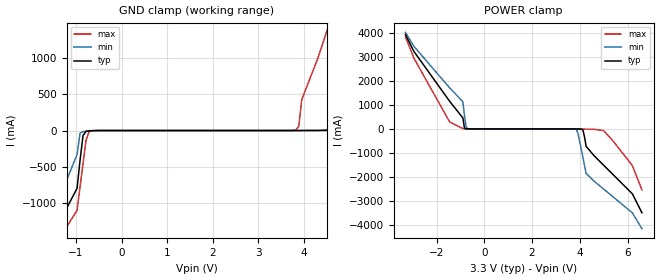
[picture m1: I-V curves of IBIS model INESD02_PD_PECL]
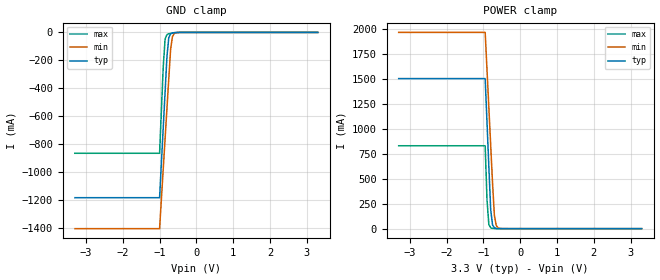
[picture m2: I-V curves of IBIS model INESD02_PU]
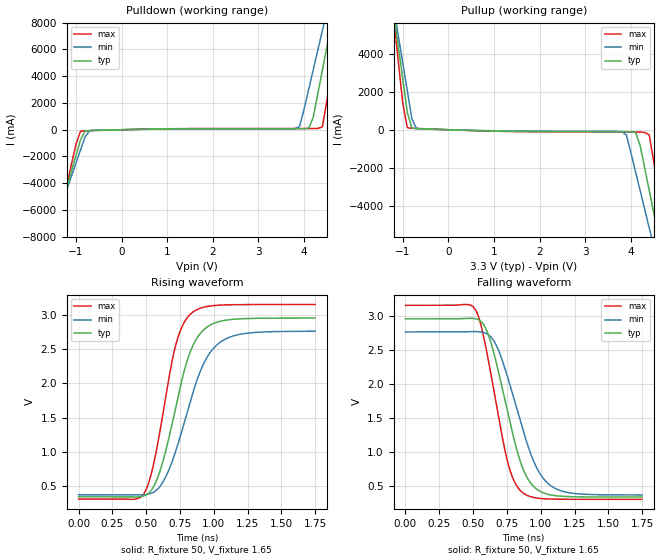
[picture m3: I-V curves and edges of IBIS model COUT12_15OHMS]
|   This file is an IBIS representation of the   |
|   Integrated Devices Technology, Inc.   |
|   ICS830584I   |
|   LOW SKEW, PCI-X 1-TO-4 FANOUT BUFFER   |
[IBIS Ver]   4.1
[File name]   830584i_3v3.ibs
[File Rev]   1.0
[Date]   2 Jun 2009 | Last modified
|   Jan  4 2007 | Generated
[Source]   Originated at Integrated Devices Technology, Inc.
[Disclaimer]
IDT hereby grants the user of this IBIS model a non-exclusive,
nontransferable license to use this IBIS model under the following terms.
Before using this IBIS model, the user should read this license.
If the user does not accept these terms,  the IBIS model should be
returned to IDT within 30 days.
   The user is granted this license only to use the IBIS model and
is not granted rights to sell, load, rent, lease or license the IBIS
model in whole or in part, or in modified form to anyone other than
user. User may modify the IBIS model to suit its specific
applications but rights to derivative works and such modifications
shall belong to IDT.
   This IBIS model is provided on an "AS IS" basis and IDT makes
absolutely no warranty with respect to the information contained
herein. IDT DISCLAIMS AND CUSTOMER WAIVES ALL WARRANTIES, EXPRESS
OR IMPLIED, INCLUDING WARRANTIES OF MERCHANTABILITY OR FITNESS FOR
A PARTICULAR PURPOSE. The entire risk as to quality and performance
is with the Customer. ACCORDINGLY, IN NO EVENT SHALL THE COMPANY BE
LIABLE FOR ANY DAMAGES, WHETHER IN CONTRACT OR TORT,INCLUDING ANY
LOST PROFITS OR OTHER INCIDENTAL, CONSEQUENTIAL, EXEMPLARY, OR
PUNITIVE DAMAGES ARISING OUT OF THE USE OR APPLICATION OF THE IBIS
model provided in this package. Further, IDT reserves the right to
make changes without notice to any product herein to improve
reliability, function, or design. IDT does not convey any license
under patent rights or any other intellectual property rights,
including those of third parties.
   IDT is not obligated to provide maintenance or support
for the licensed IBIS model.
[Copyright]   Copyright 2006 by Integrated Device Technology, Inc.
[Component]   ICS830584I
[Manufacturer] Integrated Devices Technology, Inc.
[Package]
|TSSOP 8 Lead
|   typ   min   max
R_pkg   52.5m   48.8m   56.2m
L_pkg   1.381nH   1.275nH   1.486nH
C_pkg   0.236pF   0.230pF   0.242pF
[Pin] signal_name  model_name   R_pin   L_pin   C_pin
1   CLKIN   INESD02_PD_PECL   56.2m   1.486n   0.242p
2   OE   INESD02_PU   48.8m   1.275n   0.230p
3   Q0   COUT12_15OHMS   48.8m   1.275n   0.230p
4   GND   GND   56.2m   1.468n   0.242p
5   Q1   COUT12_15OHMS   56.2m   1.486n   0.242p
6   VDD   POWER   48.8m   1.275n   0.230p
7   Q2   COUT12_15OHMS   48.8m   1.275n   0.230p
8   Q3   COUT12_15OHMS   56.2m   1.468n   0.242p
| Models and submodels in the file (3): INESD02_PD_PECL (Input), INESD02_PU (Input), COUT12_15OHMS (Output)
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[Model]   INESD02_PD_PECL
Model_type  Input
Polarity   Non-Inverting
Vinl = 0.8V
Vinh = 2.0V
|   typ   min   max
C_comp   2pF   1.5pF   2.5pF
|   typ   min   max
[Voltage range]  3.3V   3.15V   3.45V
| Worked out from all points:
|   GND clamp passes 1 mA (typ) near -0.59 V on its own axis
|   POWER clamp passes 1 mA (typ) near -0.70 V on its own axis
[GND_clamp]
-3.3V     -3.894A    -4.294A    -3.674A
-1.6V     -1.569A    -1.322A    -1.74A
-974.8mV  -794.1mA   -331.5mA   -1.096A
-843.4mV  -68.33mA   -15.34mA   -452.9mA
-646.5mV  -1.912mA   -4.151mA   -2.665mA
3.818V    89.38uA    70.49uA    7.198mA
3.95V     342.2uA    75.94uA    423.8mA
4.6V      7.437mA    165.5uA    1.553A
4.9V      78.32mA    440.9uA    2.118A
5.5V      1.293A     2.769mA    3.249A
6.25V     2.651A     112.4mA    4.38A
6.6V      3.331A     896.1mA    4.946A
[POWER_clamp]
-3.3V     3.923A     4.017A     3.838A
-2.95V    3.23A      3.44A      2.951A
-1.45V    1.149A     1.709A     289.6mA
-896.9mV  456.5mA    1.133A     15.4mA
-762.9mV  4.223mA    91.07mA    1.486mA
-695.9mV  792.2uA    10.73mA    555.6uA
3.861V    -556.7uA   -26.14mA   -39.45uA
4.129V    -41.85mA   -1.19A     -4.904mA
4.263V    -724.2mA   -1.847A    -12.04mA
5V        -1.514A    -2.505A    -71.38mA
6.2V      -2.701A    -3.492A    -1.525A
6.6V      -3.492A    -4.151A    -2.536A
[Model]   INESD02_PU
Model_type   Input
Polarity   Non-Inverting
Vinl = 0.80V
Vinh = 2.0V
|   typ   min   max
C_comp   2pF   1.5pF   2.5pF
|   typ   min   max
[Voltage range]  3.3V   3.15V   3.45V
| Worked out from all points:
|   GND clamp passes 1 mA (typ) near -0.56 V on its own axis
|   POWER clamp passes 1 mA (typ) near -0.61 V on its own axis
[GND_clamp]
|Voltage   I(typ)   I(min)   I(max)
-3.3V     -1.184A    -1.405A    -865.6mA
-1V       -1.184A    -1.405A    -865.6mA
-900mV    -678.5mA   -975.1mA   -244.1mA
-850mV    -426.2mA   -760.2mA   -46.92mA
-800mV    -174mA     -545.4mA   -16.17mA
-750mV    -37.03mA   -330.8mA   -9.981mA
-700mV    -9.767mA   -120.3mA   -7.122mA
-650mV    -3.616mA   -29.78mA   -4.922mA
-600mV    -1.7mA     -7.594mA   -3.115mA
-400mV    -123.9uA   -126uA     -173.9uA
3.3V      1.866nA    3.949uA    0A
[POWER_clamp]
|Voltage   I(typ)   I(min)   I(max)
-3.3V     1.506A     1.97A      832.1mA
-950mV    1.506A     1.97A      832.1mA
-900mV    1.063A     1.592A     287.2mA
-850mV    620.4mA    1.215A     41.77mA
-800mV    191.5mA    837.4mA    8.692mA
-750mV    37.69mA    460.1mA    3.262mA
-700mV    8.032mA    133.8mA    1.662mA
-650mV    2.005mA    32.58mA    840.1uA
-600mV    607uA      8.009mA    378.6uA
-450mV    33.11uA    139.8uA    23.88uA
3.3V      -71.13uA   -77.46uA   -62.11uA
[Model]   COUT12_15OHMS
Model_type   Output
Polarity   Non-Inverting
|   typ   min   max
C_comp   2pF   1.5pF   2.5pF
Vmeas = 1.65V
Rref = 50
Cref = 0
Vref = 1.65V
|   typ   min   max
[Voltage range]   3.3V   3.135V   3.465V
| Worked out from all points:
|   slope of the pulldown table from 0 to 0.495 V, typ, clamps not added: 13.8 ohm
|   slope of the pullup table from 0 to 0.495 V, typ, clamps not added: 13.7 ohm
|   rising waveform, R_fixture 50, V_fixture 1.65: 20-80 % time 196ps typ, 233ps min, 161ps max; typ from 0.341 V to 2.96 V
|   falling waveform, R_fixture 50, V_fixture 1.65: 20-80 % time 193ps typ, 225ps min, 163ps max; typ from 2.96 V to 0.341 V
[Pulldown]
|Voltage   I (typ)   I (min)   I (max)
-3.3V     -29.16A    -25.19A    -35.83A
-1.5V     -7.869A    -7.438A    -8.66A
-1.4V     -6.685A    -6.452A    -7.149A
-900mV    -768.5mA   -1.522A    -115.3mA
-700mV    -59.09mA   -73.31mA   -66.33mA
3.9V      79.76mA    237.3mA    91.46mA
4.2V      910.1mA    4.459A     92.62mA
4.4V      4.426A     7.39A      211.8mA
4.6V      7.945A     10.32A     4.422A
4.7V      9.706A     11.79A     6.671A
4.8V      11.47A     13.26A     8.921A
6.6V      43.31A     39.79A     49.6A
[Pullup]
|Voltage   I (typ)   I (min)   I (max)
-3.3V     43.25A     37.32A     53.22A
-1.2V     6.19A      6.441A     5.891A
-1.1V     4.426A     4.972A     3.638A
-900mV    900.3mA    2.035A     106.9mA
-700mV    58.42mA    71.68mA    66.98mA
3.8V      -101.6mA   -99.35mA   -118.6mA
4.1V      -137.6mA   -2.195A    -121.4mA
4.3V      -1.989A    -4.161A    -136.8mA
4.4V      -3.169A    -5.144A    -265.7mA
4.6V      -5.53A     -7.113A    -3.183A
4.8V      -7.892A    -9.082A    -6.199A
6.6V      -29.16A    -26.81A    -33.35A
[Ramp]
|   typ   min   max
dV/dt_r   2.093/0.305n   1.914/0.364n   2.279/0.249n
dV/dt_f   2.098/0.289n   1.918/0.339n   2.286/0.243n
R_load =   50.0000
[Rising Waveform]
R_fixture = 50
V_fixture = 1.65   |Vcc_typ
V_fixture_min = 1.5675 |Vcc_min
V_fixture_max = 1.7325 |Vcc_max
C_fixture = 0.0p
| Time   typ   min   max
0s        340.7mV    370.7mV    307.4mV
487ps     357.9mV    371.6mV    399.2mV
537.8ps   436.5mV    393.1mV    680.8mV
593.8ps   670.5mV    472.7mV    1.213V
718.2ps   1.65V      1.01V      2.56V
770.8ps   2.104V     1.354V     2.855V
837.3ps   2.518V     1.812V     3.031V
947.7ps   2.821V     2.374V     3.124V
1.083ns   2.922V     2.645V     3.147V
1.748ns   2.955V     2.762V     3.153V
[Falling Waveform]
R_fixture = 50
V_fixture = 1.65   |Vcc_typ
V_fixture_min = 1.5675 |Vcc_min
V_fixture_max = 1.7325 |Vcc_max
C_fixture = 0.0p
| Time   typ   min   max
0s        2.955V     2.763V     3.153V
515ps     2.957V     2.769V     3.095V
551.8ps   2.927V     2.764V     2.909V
593.8ps   2.814V     2.743V     2.543V
670.9ps   2.315V     2.569V     1.715V
767.3ps   1.49V      2.021V     771.3mV
865.4ps   772.6mV    1.349V     407mV
975.7ps   448.5mV    748.1mV    324.9mV
1.098ns   363.7mV    476.5mV    310.5mV
1.748ns   340.8mV    371.1mV    307.4mV
